| IBIS file was generated by Viper version: 2022.06.14
[IBIS Ver]   4.2
[Comment Char]   |_char
[File Name]   ke17z512_100lqfp14x14.ibs
[File Rev]   1
[Date]   Tue Jun 27 20:49:57 2023
[Source]   NXP Viper 2022.06.14
[Notes]
[Disclaimer] IMPORTANT NOTICE
  This information is provided on an AS IS basis and without warranty.
  IN NO EVENT SHALL NXP BE LIABLE FOR INCIDENTAL OR CONSEQUENTIAL
  DAMAGES ARISING FROM USE OF THIS INFORMATION. THIS DISCLAIMER OF
  WARRANTY EXTENDS TO THE USER OF THE INFORMATION, AND TO THEIR CUSTOMERS
  OR USERS OF PRODUCTS  AND IS IN LIEU OF ALL WARRANTIES WHETHER EXPRESS,
  IMPLIED, OR STATUTORY, INCLUDING IMPLIED WARRANTIES OF MERCHANTABILITY
  OR FITNESS FOR PARTICULAR PURPOSE.
  NXP does not represent or warrant that the information furnished
  hereunder is free of infringement of any third party patents,
  copyrights, trade secrets, or other intellectual property rights.
  NXP does not represent or warrant that the information is free of
  defect, or that it meets any particular standard, requirements or need
  of the user of the infomation or their customers.
  NXP reserves the right to change the information in this file
  without notice.
   http://www.nxp.com
[Copyright]   (C) Copyright NXP 2004 - 2023, All Rights Reserved.
|   KE17Z512_100LQFP14x14
[Component]   KE17Z512_100LQFP14x14
[Manufacturer]   NXP
[Package]
| variable   typ   min   max
R_pkg   0.24824   0.14526   0.28043
L_pkg   6.312e-09   5.223e-09   8.666e-09
C_pkg   3.403e-13   2.687e-13   3.122e-12
[Pin] signal_name   model_name   R_pin   L_pin   C_pin
1   PTE16   p_io_5ma_model   0.27108   7.053e-09 3.329e-13
2   PTE15   p_io_5ma_model   0.26547   6.711e-09 3.376e-13
3   PTD1   p_io_20ma_model   0.26314   6.509e-09 3.294e-13
4   PTD0   p_io_20ma_model   0.1542   5.686e-09 3.806e-13
5   PTE11   p_io_5ma_model   0.26136   6.317e-09 3.184e-13
6   PTE10   p_io_5ma_model   0.25821   6.195e-09 3.132e-13
7   PTE13   p_io_5ma_model   0.25681   6.051e-09 3.075e-13
8   PTE5   p_io_5ma_model   0.2569   5.925e-09 3.011e-13
9   PTE4   p_io_5ma_model   0.25862   5.688e-09 2.947e-13
10   VDD   POWER   NA   NA   NA
11   VDDA   POWER   NA   NA   NA
12   VREFH   POWER   0.27322   5.736e-09 2.793e-13
13   VREFL   GND   0.27482   5.918e-09 2.792e-13
14   VSS   GND   NA   NA   NA
15   PTB7   p_io_5ma_model   0.26204   5.786e-09 2.808e-13
16   PTB6   p_io_5ma_model   0.25601   5.920e-09 2.882e-13
17   PTE14   p_io_5ma_model   0.25285   5.957e-09 2.936e-13
18   PTE3   p_io_5ma_model   0.25134   6.009e-09 2.982e-13
19   PTE12   p_io_5ma_model   0.251   6.055e-09 3.034e-13
20   PTD17   p_io_5ma_model   0.25164   6.109e-09 3.067e-13
21   PTD16   p_io_20ma_model   0.26265   6.405e-09 3.025e-13
22   PTD15   p_io_20ma_model   0.25489   6.234e-09 3.192e-13
23   PTE9   p_io_5ma_model   0.15105   5.619e-09 3.832e-13
24   PTD14   p_io_5ma_model   0.25718   6.394e-09 3.252e-13
25   PTD13   p_io_5ma_model   0.26623   6.617e-09 3.242e-13
26   PTE8   p_io_5ma_model   0.26783   6.608e-09 3.334e-13
27   PTB5   p_io_20ma_model   0.2636   6.459e-09 3.382e-13
28   PTB4   p_io_20ma_model   0.15437   5.791e-09 3.859e-13
29   PTC3   p_io_5ma_model   0.25983   6.302e-09 3.262e-13
30   PTC2   p_io_5ma_model   0.25512   6.209e-09 3.169e-13
31   PTD7   p_io_5ma_model   0.25174   6.093e-09 3.095e-13
32   PTD6   p_io_5ma_model   0.25024   6.016e-09 3.024e-13
33   PTD5   p_io_5ma_model   0.24924   5.940e-09 2.970e-13
34   PTD12   p_io_5ma_model   0.2496   5.883e-09 2.905e-13
35   PTD11   p_io_5ma_model   0.25169   5.797e-09 2.838e-13
36   PTD10   p_io_5ma_model   0.25759   5.660e-09 2.776e-13
37   VSS   GND   NA   NA   NA
38   VDD   POWER   NA   NA   NA
39   PTC1   p_io_5ma_model   0.16537   5.223e-09 3.206e-13
40   PTC0   p_io_5ma_model   0.25307   5.813e-09 2.761e-13
41   PTD9   p_io_5ma_model   0.24649   5.822e-09 2.808e-13
42   PTD8   p_io_5ma_model   0.24351   5.833e-09 2.840e-13
43   PTC17   p_io_5ma_model   0.24252   5.871e-09 2.902e-13
44   PTC16   p_io_5ma_model   0.14526   5.342e-09 3.480e-13
45   PTC15   p_io_5ma_model   0.24147   5.973e-09 3.013e-13
46   PTC14   p_io_5ma_model   0.25212   6.301e-09 2.980e-13
47   PTB3   p_io_5ma_model   0.24408   6.159e-09 3.094e-13
48   PTB2   p_io_10ma_model   0.24616   6.251e-09 3.172e-13
49   PTC13   p_io_5ma_model   0.25044   6.373e-09 3.233e-13
50   PTC12   p_io_5ma_model   0.26255   6.590e-09 3.238e-13
51   PTC11   p_io_5ma_model   0.26909   6.688e-09 3.334e-13
52   PTC10   p_io_5ma_model   0.26394   6.522e-09 3.375e-13
53   PTB1   p_io_5ma_model   0.25972   6.372e-09 3.289e-13
54   PTB0   p_io_5ma_model   0.25682   6.246e-09 3.206e-13
55   PTC9   p_io_5ma_model   0.25468   6.126e-09 3.130e-13
56   PTC8   p_io_5ma_model   0.25456   6.002e-09 3.102e-13
57   PTA7   p_io_5ma_model   0.15118   5.313e-09 3.606e-13
58   PTA6   p_io_5ma_model   0.25571   5.787e-09 3.023e-13
59   PTE7   p_io_5ma_model   0.25779   5.589e-09 2.947e-13
60   VSS   GND   NA   NA   NA
61   VDD   POWER   NA   NA   NA
62   PTA17   p_io_5ma_model   0.27366   5.896e-09 2.815e-13
63   PTB17   p_io_5ma_model   0.2721   6.129e-09 2.799e-13
64   PTB16   p_io_5ma_model   0.26609   6.125e-09 2.790e-13
65   PTB15   p_io_5ma_model   0.25831   6.083e-09 2.836e-13
66   PTB14   p_io_10ma_model   0.25382   6.045e-09 2.847e-13
67   PTB13   p_io_5ma_model   0.25086   6.028e-09 2.896e-13
68   PTB12   p_io_5ma_model   0.24944   6.048e-09 2.973e-13
69   PTD4   p_io_5ma_model   0.24911   6.088e-09 3.026e-13
70   PTD3   p_io_rst_model   0.24981   6.161e-09 3.079e-13
71   PTD2   p_io_5ma_model   0.26199   6.513e-09 3.041e-13
72   PTA3   p_io_5ma_model   0.25461   6.306e-09 3.183e-13
73   PTA2   p_io_5ma_model   0.1509   5.697e-09 3.823e-13
74   PTB11   p_io_5ma_model   0.25693   6.435e-09 3.260e-13
75   PTB10   p_io_5ma_model   0.26792   6.758e-09 3.258e-13
76   PTB9   p_io_5ma_model   0.28043   8.508e-09 3.333e-13
77   PTB8   p_io_5ma_model   0.27442   8.185e-09 3.376e-13
78   PTA1   p_io_5ma_model   0.26931   7.916e-09 3.280e-13
79   PTA0   p_io_5ma_model   0.26559   7.648e-09 3.190e-13
80   PTC7   p_io_5ma_model   0.26257   7.409e-09 3.108e-13
81   PTC6   p_io_5ma_model   0.26033   7.162e-09 3.064e-13
82   PTA16   p_io_5ma_model   0.25898   6.923e-09 3.003e-13
83   PTA15   p_io_5ma_model   0.25872   6.658e-09 2.937e-13
84   PTE6   p_io_5ma_model   0.25988   6.293e-09 2.859e-13
85   PTE2   p_io_5ma_model   0.26565   5.863e-09 2.798e-13
86   VSS   GND   NA   NA   NA
87   VDD   POWER   NA   NA   NA
88   PTA14   p_io_5ma_model   0.27007   5.853e-09 2.687e-13
89   PTA13   p_io_5ma_model   0.25928   5.935e-09 2.687e-13
90   PTA12   p_io_5ma_model   0.24982   5.847e-09 2.759e-13
91   PTA11   p_io_5ma_model   0.14843   5.241e-09 3.122e-12
92   PTA10   p_io_5ma_model   0.24314   5.921e-09 2.828e-13
93   PTE1   p_io_20ma_model   0.24176   6.207e-09 2.852e-13
94   PTE0   p_io_20ma_model   0.24248   6.511e-09 2.937e-13
95   PTC5   p_io_5ma_model   0.24458   6.831e-09 3.015e-13
96   PTC4   p_io_5ma_model   0.24766   7.158e-09 3.023e-13
97   PTA5   p_io_rst_model   0.24964   7.471e-09 3.077e-13
98   PTA4   p_io_5ma_model   0.25358   7.826e-09 3.191e-13
99   PTA9   p_io_5ma_model   0.25888   8.202e-09 3.225e-13
100   PTA8   p_io_5ma_model   0.2706   8.666e-09 3.216e-13
[Pin Mapping]   pulldown_ref   pullup_ref
1   VSS   VDD
2   VSS   VDD
3   VSS   VDD
4   VSS   VDD
5   VSS   VDD
6   VSS   VDD
7   VSS   VDD
8   VSS   VDD
9   VSS   VDD
10   NC   VDD
11   NC   VDDA
12   NC   VREFH
13   VREFL   NC
14   VSS   NC
15   VSS   VDD
16   VSS   VDD
17   VSS   VDD
18   VSS   VDD
19   VSS   VDD
20   VSS   VDD
21   VSS   VDD
22   VSS   VDD
23   VSS   VDD
24   VSS   VDD
25   VSS   VDD
26   VSS   VDD
27   VSS   VDD
28   VSS   VDD
29   VSS   VDD
30   VSS   VDD
31   VSS   VDD
32   VSS   VDD
33   VSS   VDD
34   VSS   VDD
35   VSS   VDD
36   VSS   VDD
37   VSS   NC
38   NC   VDD
39   VSS   VDD
40   VSS   VDD
41   VSS   VDD
42   VSS   VDD
43   VSS   VDD
44   VSS   VDD
45   VSS   VDD
46   VSS   VDD
47   VSS   VDD
48   VSS   VDD
49   VSS   VDD
50   VSS   VDD
51   VSS   VDD
52   VSS   VDD
53   VSS   VDD
54   VSS   VDD
55   VSS   VDD
56   VSS   VDD
57   VSS   VDD
58   VSS   VDD
59   VSS   VDD
60   VSS   NC
61   NC   VDD
62   VSS   VDD
63   VSS   VDD
64   VSS   VDD
65   VSS   VDD
66   VSS   VDD
67   VSS   VDD
68   VSS   VDD
69   VSS   VDD
70   VSS   VDD
71   VSS   VDD
72   VSS   VDD
73   VSS   VDD
74   VSS   VDD
75   VSS   VDD
76   VSS   VDD
77   VSS   VDD
78   VSS   VDD
79   VSS   VDD
80   VSS   VDD
81   VSS   VDD
82   VSS   VDD
83   VSS   VDD
84   VSS   VDD
85   VSS   VDD
86   VSS   NC
87   NC   VDD
88   VSS   VDD
89   VSS   VDD
90   VSS   VDD
91   VSS   VDD
92   VSS   VDD
93   VSS   VDD
94   VSS   VDD
95   VSS   VDD
96   VSS   VDD
97   VSS   VDD
98   VSS   VDD
99   VSS   VDD
100   VSS   VDD
|*   Model Selector   *
[Model Selector] p_io_10ma_model
p_io_3p3_10ma_ds0   half-drive for 3.3v application
p_io_3p3_10ma_ds1   full-drive for 3.3v application
p_io_5p0_10ma_ds0   half-drive for 5.0v application
p_io_5p0_10ma_ds1   full-drive for 5.0v application
[Model Selector] p_io_20ma_model
p_io_3p3_20ma_ds0   half-drive for 3.3v application
p_io_3p3_20ma_ds1   full-drive for 3.3v application
p_io_5p0_20ma_ds0   half-drive for 5.0v application
p_io_5p0_20ma_ds1   full-drive for 5.0v application
[Model Selector] p_io_5ma_model
p_io_3p3_5ma   for 3.3v application
p_io_5p0_5ma   for 5.0v application
[Model Selector] p_io_rst_model
p_io_3p3_rst   for 3.3v application
p_io_5p0_rst   for 5.0v application
| End [Component] MT512X_100LQFP14x14
| Models and submodels in the file (12): p_io_3p3_10ma_ds0 (I/O), p_io_3p3_10ma_ds1 (I/O), p_io_3p3_20ma_ds0 (I/O), p_io_3p3_20ma_ds1 (I/O), p_io_3p3_5ma (I/O), p_io_3p3_rst (I/O), p_io_5p0_10ma_ds0 (I/O), p_io_5p0_10ma_ds1 (I/O), p_io_5p0_20ma_ds0 (I/O), p_io_5p0_20ma_ds1 (I/O), p_io_5p0_5ma (I/O), p_io_5p0_rst (I/O)
